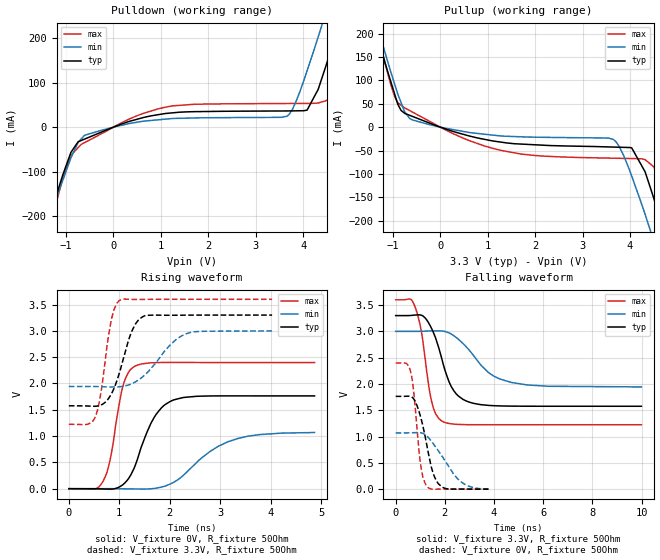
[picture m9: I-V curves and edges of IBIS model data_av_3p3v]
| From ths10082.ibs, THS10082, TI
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|   data_av_3p3v Model
[Model]   data_av_3p3v
Model_type   Output
Polarity   Non-Inverting
Vmeas = 1.65
Vref = 1.65
Cref = 2pF
Rref = 50
|   typ   min   max
C_comp   1.935e-12   1.924e-12   1.989e-12
[Voltage Range]   3.3   3   3.6
|Ambient Temperature   25   85   -40
|Junction Temperature
[Temperature Range]   27   125   -40
[Pullup Reference]   3.3   3   3.6
[Pulldown Reference]   0   0   0
[Power Clamp Reference]   3.3   3   3.6
[GND Clamp Reference]   0   0   0
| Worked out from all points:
|   slope of the pulldown table from 0 to 0.495 V, typ, clamps not added: 28 ohm
|   slope of the pullup table from 0 to 0.495 V, typ, clamps not added: 31.6 ohm
|   falling waveform, V_fixture 3.3V, R_fixture 50Ohm: 20-80 % time 745ps typ, 1.28ns min, 455ps max; typ from 3.3 V to 1.58 V
|   rising waveform, V_fixture 0V, R_fixture 50Ohm: 20-80 % time 454ps typ, 850ps min, 263ps max; typ from 0 V to 1.76 V
|   rising waveform, V_fixture 3.3V, R_fixture 50Ohm: 20-80 % time 332ps typ, 575ps min, 213ps max; typ from 1.58 V to 3.3 V
|   falling waveform, V_fixture 0V, R_fixture 50Ohm: 20-80 % time 501ps typ, 943ps min, 295ps max; typ from 1.76 V to 0 V
[Pulldown]
|   Voltage   I(typ)   I(min)   I(max)
-3.3V     -973.3mA   -899.3mA   -1.066A
-1.426V   -232.9mA   -231.2mA   -257.5mA
-897.6mV  -57.05mA   -69.51mA   -63.83mA
-591mV    -26.14mA   -17.74mA   -33.87mA
1.091V    30.64mA    17.96mA    44.81mA
3.66V     36.44mA    24.72mA    53.22mA
4.082V    38.22mA    126.7mA    53.44mA
4.316V    84.92mA    202.9mA    54.32mA
4.468V    133.9mA    254.5mA    59.08mA
4.684V    211.3mA    330.4mA    106mA
5.13V     373.7mA    488.7mA    269.1mA
6.6V      940.4mA    1.035A     855.6mA
[Pullup]
|   Voltage   I(typ)   I(min)   I(max)
-3.3V     979.6mA    958.6mA    1.018A
-1.39V    222.2mA    239.6mA    223.9mA
-961.2mV  70.15mA    91.45mA    64.82mA
-828.3mV  35.79mA    52.8mA     47.13mA
-591mV    23.07mA    15.51mA    32.43mA
1.246V    -31.57mA   -18.56mA   -49.05mA
3.645V    -42.63mA   -26.18mA   -66.44mA
4.036V    -44.49mA   -104.9mA   -67.21mA
4.468V    -141.8mA   -233.5mA   -82.15mA
4.709V    -224.2mA   -313.6mA   -144.8mA
4.867V    -279mA     -367mA     -205.6mA
6.6V      -956.8mA   -986.6mA   -929.7mA
[Ramp]
R_load = 50
|   typ   min   max
dV/dt_r   1.05825/4.52692e-10   0.642047/8.45553e-10   1.43893/2.61746e-10
dV/dt_f   1.0345/7.40402e-10   0.633811/1.27322e-09   1.42541/4.53882e-10
[Falling Waveform]
V_fixture = 3.3V
V_fixture_min = 3V
V_fixture_max = 3.6V
R_fixture = 50Ohm
|   Time   V(typ)   V(min)   V(max)
0s        3.3V       3V         3.6V
784ps     3.31V      3V         3.471V
1.054ns   3.306V     3.001V     2.976V
1.458ns   3.057V     3.009V     1.675V
1.864ns   2.5V       3.008V     1.299V
2.364ns   1.871V     2.917V     1.237V
3.184ns   1.629V     2.53V      1.225V
3.776ns   1.592V     2.216V     1.224V
4.714ns   1.578V     2.028V     1.224V
9.998ns   1.576V     1.944V     1.224V
[Rising Waveform]
V_fixture = 0V
V_fixture_min = 0V
V_fixture_max = 0V
R_fixture = 50Ohm
|   Time   V(typ)   V(min)   V(max)
0s        1.442nV    2.279nV    1.234nV
514ps     -1.132mV   195.7uV    -8.795mV
680ps     -5.568mV   229.6uV    143.7mV
832ps     -8.38mV    -132.3uV   611.8mV
1.074ns   78.06mV    -2.154mV   1.953V
1.314ns   437.5mV    -5.4mV     2.332V
1.692ns   1.356V     3.821mV    2.394V
2.076ns   1.687V     120mV      2.4V
3.142ns   1.764V     887.5mV    2.398V
4.87ns    1.764V     1.068V     2.398V
[Rising Waveform]
V_fixture = 3.3V
V_fixture_min = 3V
V_fixture_max = 3.6V
R_fixture = 50Ohm
|   Time   V(typ)   V(min)   V(max)
0s        1.576V     1.943V     1.224V
524ps     1.567V     1.942V     1.363V
628ps     1.587V     1.939V     1.778V
840ps     1.796V     1.933V     3.194V
1.004ns   2.206V     1.937V     3.579V
1.25ns    2.995V     1.996V     3.598V
1.5ns     3.286V     2.157V     3.598V
2.016ns   3.296V     2.739V     3.6V
2.394ns   3.299V     2.966V     3.6V
4.028ns   3.3V       2.999V     3.6V
[Falling Waveform]
V_fixture = 0V
V_fixture_min = 0V
V_fixture_max = 0V
R_fixture = 50Ohm
|   Time   V(typ)   V(min)   V(max)
0s        1.764V     1.07V      2.398V
428ps     1.766V     1.07V      2.391V
616ps     1.761V     1.071V     2.218V
732ps     1.717V     1.073V     1.856V
998ps     1.399V     1.074V     527.3mV
1.232ns   921mV      1.023V     80.97mV
1.528ns   297.3mV    863.9mV    1.689mV
1.86ns    47.8mV     645mV      659.6uV
2.63ns    1.711mV    149.2mV    163uV
3.776ns   230.9uV    2.765mV    130.2uV
